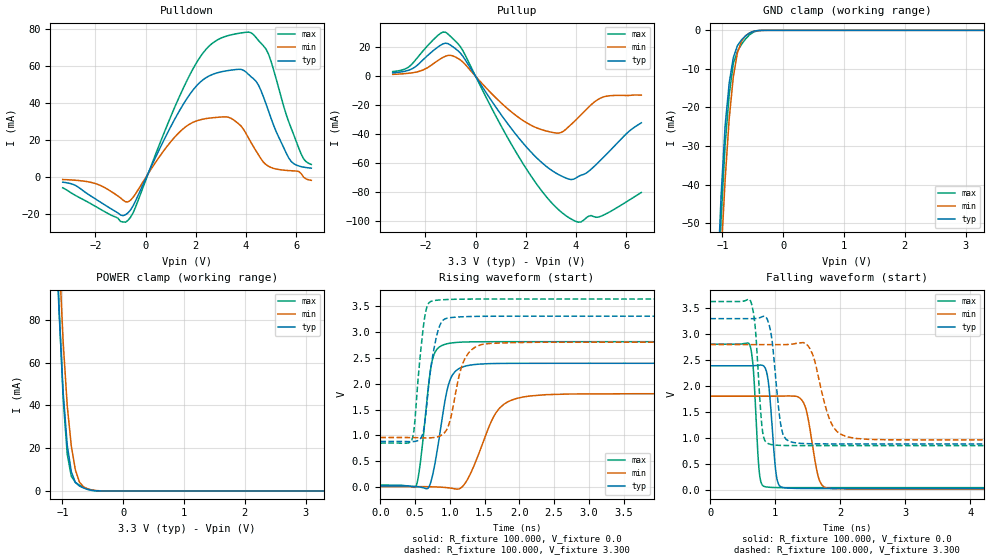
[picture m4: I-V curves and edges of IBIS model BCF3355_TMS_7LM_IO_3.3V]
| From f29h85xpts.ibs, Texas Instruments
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|BCF3355_TMS_7LM_IO_3.3V;
|   Model BCF3355_TMS_7LM_IO_3.3V
[Model]   BCF3355_TMS_7LM_IO_3.3V
Model_type   I/O
Polarity   Non-Inverting
Enable   Active-Low
Vinl =   0.800V
Vinh =   2.000V
Vmeas =  1.650V
Cref =   15.000pF
Vref =   0.0V
|   typ   min   max
C_comp   0.768pF   0.760pF   0.835pF
[Model Spec]
Vinh   2.000V   2.000V   2.000V
Vinl   0.800V   0.800V   0.800V
[Temperature Range]   25   155   -40
[Voltage Range]   3.300V   2.800V   3.630V
[Pullup Reference]   3.300V   2.800V   3.630V
[Pulldown Reference]   0.0V   0.0V   0.0V
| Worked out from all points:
|   slope of the pulldown table from 0 to 0.495 V, typ, clamps not added: 34.2 ohm
|   slope of the pullup table from 0 to 0.495 V, typ, clamps not added: 37 ohm
|   GND clamp passes 1 mA (typ) near -0.58 V on its own axis
|   POWER clamp passes 1 mA (typ) near -0.62 V on its own axis
|   rising waveform, R_fixture 100.000, V_fixture 0.0: 20-80 % time 177ps typ, 335ps min, 135ps max; typ from 0.026 V to 2.39 V
|   rising waveform, R_fixture 100.000, V_fixture 3.300: 20-80 % time 143ps typ, 190ps min, 113ps max; typ from 0.885 V to 3.3 V
|   falling waveform, R_fixture 100.000, V_fixture 0.0: 20-80 % time 88.4ps typ, 147ps min, 71ps max; typ from 2.39 V to 0.026 V
|   falling waveform, R_fixture 100.000, V_fixture 3.300: 20-80 % time 115ps typ, 230ps min, 86.3ps max; typ from 3.3 V to 0.885 V
[Pulldown]
|Voltage   I(typ)   I(min)   I(max)
-3.3V     -2.79mA    -1.345mA   -5.802mA
-2V       -11.81mA   -3.512mA   -15.83mA
-700mV    -19.38mA   -13.44mA   -23.4mA
1.1V      29.74mA    20.65mA    35.82mA
2.1V      50.32mA    30.67mA    63.38mA
3.3V      57.6mA     32.33mA    76.51mA
4V        56.76mA    23.55mA    78.28mA
4.5V      49.61mA    11.95mA    73.76mA
4.8V      39.39mA    6.682mA    69.08mA
5.7V      10.32mA    3.491mA    29.9mA
6.3V      5.341mA    -156.7uA   9.702mA
6.6V      4.794mA    -1.775mA   6.818mA
[Pullup]
|Voltage   I(typ)   I(min)   I(max)
-3.3V     2.421mA    1.372mA    3.294mA
-2.7V     4.051mA    2.079mA    6.053mA
-1.5V     20.35mA    10.98mA    28.39mA
-1.1V     22.68mA    14.51mA    29.35mA
-500mV    13.8mA     9.799mA    17.64mA
1V        -26.15mA   -18.12mA   -33.81mA
2.1V      -50.45mA   -32.85mA   -66.24mA
3.3V      -68.04mA   -39.35mA   -92.37mA
3.8V      -71.55mA   -33.42mA   -98.84mA
4.1V      -69.33mA   -28.38mA   -101.1mA
5V        -57.73mA   -14.86mA   -96.93mA
6.6V      -32.2mA    -13.02mA   -80.5mA
[GND_clamp]
|Voltage   I(typ)   I(min)   I(max)
-3.3V     -1.224A    -1.023A    -1.58A
-1.089V   -67.9mA    -81.11mA   -78.84mA
-1.022V   -42.88mA   -58.51mA   -48.94mA
-955mV    -24.63mA   -38.63mA   -29.53mA
-888mV    -13.58mA   -22.81mA   -16.65mA
-821mV    -7.1mA     -12.08mA   -8.623mA
-754mV    -3.998mA   -5.899mA   -5.406mA
-687mV    -2.49mA    -2.853mA   -3.663mA
-620mV    -1.44mA    -1.429mA   -2.253mA
-553mV    -678.6uA   -680.7uA   -1.15mA
-352mV    -7.12uA    -20.42uA   -18.15uA
3.3V      0A         0A         0A
[POWER_clamp]
|Voltage   I(typ)   I(min)   I(max)
-3.3V     2.006A     2.26A      2.214A
-1.122V   128.5mA    158.7mA    137.5mA
-1.055V   83.49mA    110.3mA    86.09mA
-988mV    46.07mA    69.65mA    43.21mA
-921mV    21.4mA     39.86mA    17.15mA
-854mV    9mA        21.02mA    6.849mA
-787mV    3.925mA    9.835mA    4.009mA
-720mV    2.286mA    4.115mA    2.69mA
-653mV    1.377mA    1.896mA    1.611mA
-586mV    710.7uA    988.8uA    774.2uA
-385mV    15.51uA    61.71uA    9.433uA
3.3V      0A         0A         0A
[Ramp]
| variable   typ   min   max
dV/dt_r   1.419/0.178n   1.075/0.335n   1.659/0.135n
dV/dt_f   1.448/0.115n   1.103/0.229n   1.665/85.982p
R_load = 100.000
[Rising Waveform]
R_fixture= 100.000
V_fixture= 0.0
V_fixture_min= 0.0
V_fixture_max= 0.0
|time   V(typ)   V(min)   V(max)
0s        25.76mV    13.39mV    42.38mV
517ps     15.76mV    14.32mV    33.38mV
582ps     3.279mV    14.27mV    534.4mV
683ps     -20.19mV   12.85mV    1.828V
750ps     221.4mV    10.66mV    2.458V
971ps     1.928V     -6.911mV   2.77V
1.226ns   2.337V     89.53mV    2.801V
1.717ns   2.388V     1.529V     2.807V
2.147ns   2.39V      1.76V      2.807V
10ns      2.391V     1.805V     2.807V
[Rising Waveform]
R_fixture= 100.000
V_fixture= 3.300
V_fixture_min= 2.800
V_fixture_max= 3.630
|time   V(typ)   V(min)   V(max)
0s        884.8mV    960.7mV    853mV
454ps     881.2mV    959.5mV    915.2mV
486ps     884.3mV    958.9mV    1.119V
617ps     1.061V     954.8mV    3.06V
674ps     1.664V     953.6mV    3.488V
753ps     2.526V     957.8mV    3.594V
907ps     3.225V     1.029V     3.616V
1.196ns   3.288V     2.416V     3.627V
1.463ns   3.296V     2.754V     3.628V
10ns      3.298V     2.799V     3.628V
[Falling Waveform]
R_fixture= 100.000
V_fixture= 0.0
V_fixture_min= 0.0
V_fixture_max= 0.0
|time   V(typ)   V(min)   V(max)
0s        2.391V     1.805V     2.807V
607ps     2.391V     1.804V     2.795V
666ps     2.392V     1.804V     2.266V
760ps     2.402V     1.804V     275.9mV
846ps     2.344V     1.804V     60.01mV
1.016ns   280.4mV    1.805V     44.33mV
1.128ns   41.64mV    1.807V     42.88mV
1.435ns   27.11mV    1.678V     42.34mV
1.799ns   26.1mV     33.63mV    42.32mV
10ns      25.71mV    13.39mV    42.32mV
[Falling Waveform]
R_fixture= 100.000
V_fixture= 3.300
V_fixture_min= 2.800
V_fixture_max= 3.630
|time   V(typ)   V(min)   V(max)
0s        3.298V     2.799V     3.628V
621ps     3.297V     2.799V     3.634V
689ps     3.299V     2.799V     3.165V
804ps     3.337V     2.799V     1.123V
935ps     3.004V     2.799V     874.1mV
1.089ns   1.221V     2.798V     856.5mV
1.273ns   913.8mV    2.809V     853.5mV
1.903ns   885.3mV    1.192V     852.9mV
2.243ns   885mV      990.6mV    852.9mV
10ns      884.7mV    960.7mV    852.9mV
